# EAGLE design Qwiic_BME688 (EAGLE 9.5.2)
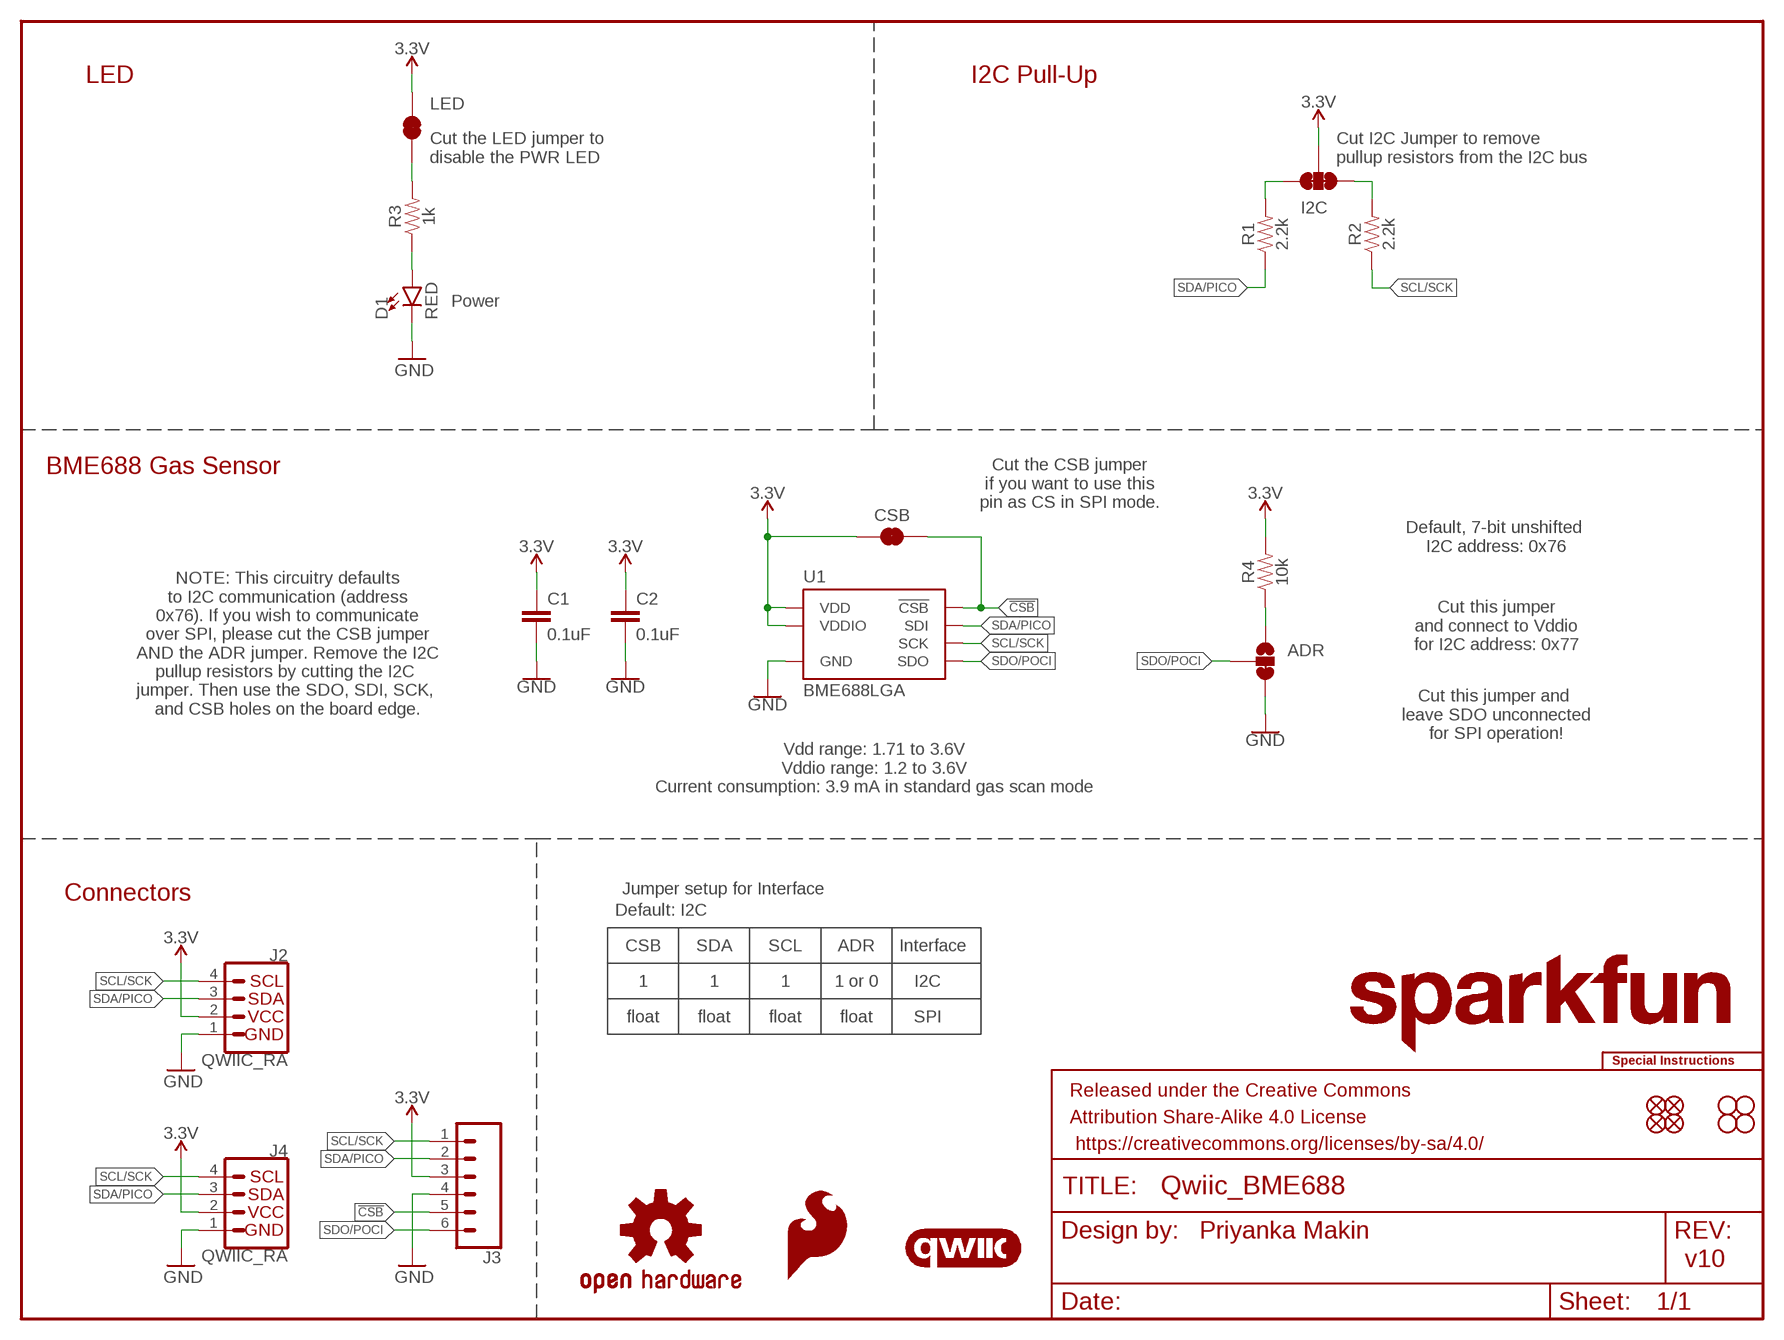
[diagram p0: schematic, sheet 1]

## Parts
ADR  JUMPER-SMT_3_1-NC_TRACE_SILK  [SMT-JUMPER_3_1-NC_TRACE_SILK]
C1  0.1uF  0.1UF-0603-100V-10%  [0603]
C2  0.1uF  0.1UF-0603-100V-10%  [0603]
CSB  JUMPER-SMT_2_NC_TRACE_SILK  [SMT-JUMPER_2_NC_TRACE_SILK]
D1  RED  LED-RED0603  [LED-0603]
FRAME1  FRAME-LETTER  [CREATIVE_COMMONS]
I2C  JUMPER-SMT_3_2-NC_TRACE_SILK  [SMT-JUMPER_3_2-NC_TRACE_SILK]
J2  QWIIC_RA  QWIIC_CONNECTORJS-1MM  [JST04_1MM_RA]
J3  CONN_06NO_SILK_NO_POP  [1X06_NO_SILK]
J4  QWIIC_RA  QWIIC_CONNECTORJS-1MM  [JST04_1MM_RA]
JP1  FIDUCIALUFIDUCIAL  [FIDUCIAL-MICRO]
JP2  FIDUCIALUFIDUCIAL  [FIDUCIAL-MICRO]
JP3  STAND-OFF  [STAND-OFF]
JP4  STAND-OFF  [STAND-OFF]
JP5  FIDUCIALUFIDUCIAL  [FIDUCIAL-MICRO]
JP6  FIDUCIALUFIDUCIAL  [FIDUCIAL-MICRO]
JP7  STAND-OFF  [STAND-OFF]
JP8  STAND-OFF  [STAND-OFF]
LED  JUMPER-SMT_2_NC_TRACE_SILK  [SMT-JUMPER_2_NC_TRACE_SILK]
LOGO1  SPECIAL_INSTRUCTIONS-ORDERING  [ORDERING_INSTRUCTIONS]
LOGO2  QWIIC_LOGO_5MM  [QWIIC_5MM]
LOGO3  SFE_LOGO_NAME.1_INCH  [SFE_LOGO_NAME_.1]
LOGO4  SFE_LOGO_FLAME.1_INCH  [SFE_LOGO_FLAME_.1]
LOGO5  OSHW-LOGOS  [OSHW-LOGO-S]
LOGO6  SFE_LOGO_NAME.1_INCH  [SFE_LOGO_NAME_.1]
R1  2.2k  2.2KOHM-0603-1/10W-1%  [0603]
R2  2.2k  2.2KOHM-0603-1/10W-1%  [0603]
R3  1k  1KOHM-0603-1/10W-1%  [0603]
R4  10k  10KOHM-0603-1/10W-1%  [0603]
U1  BME688LGA  [LGA_8PIN]

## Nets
3.3V: C1.1 C2.1 CSB.1 I2C.2 J2.2 J3.3 J4.2 LED.2 R4.2 U1.6(VDDIO) U1.8(VDD)
!CSB!: CSB.2 J3.5 U1.2(!CSB!)
GND: ADR.3 C1.2 C2.2 D1.C J2.1 J3.4 J4.1 U1.1(GND) U1.7(GND)
N$1: LED.1 R3.2
N$2: I2C.3 R1.2
N$3: D1.A R3.1
N$4: I2C.1 R2.2
N$5: ADR.1 R4.1
SCL/SCK: J2.4 J3.1 J4.4 R2.1 U1.4(SCK)
SDA/PICO: J2.3 J3.2 J4.3 R1.1 U1.3(SDI)
SDO/POCI: ADR.2 J3.6 U1.5(SDO)

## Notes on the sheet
- LED | I2C Pull-Up
- Cut the LED jumper to
  disable the PWR LED
- Cut I2C Jumper to remove 
  pullup resistors from the I2C bus
- Power
- BME688 Gas Sensor
- Cut the CSB jumper
  if you want to use this
  pin as CS in SPI mode.
- Default, 7-bit unshifted 
  I2C address: 0x76
- Cut this jumper
  and connect to Vddio
  for I2C address: 0x77
- NOTE: This circuitry defaults
  to I2C communication (address
  0x76). If you wish to communicate
  over SPI, please cut the CSB jumper
  AND the ADR jumper. Remove the I2C
  pullup resistors by cutting the I2C 
  jumper. Then use the SDO, SDI, SCK, 
  and CSB holes on the board edge.
- Cut this jumper and 
  leave SDO unconnected
  for SPI operation!
- Vdd range: 1.71 to 3.6V
  Vddio range: 1.2 to 3.6V
  Current consumption: 3.9 mA in standard gas scan mode
- Connectors | Jumper setup for Interface
- Default: I2C
- CSB | SDA | SCL | ADR | Interface
- 1 | 1 | 1 | 1 or 0 | I2C
- float | float | float | float | SPI
- Priyanka Makin
- v10

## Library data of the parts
ADR = SparkFun-Jumpers:JUMPER-SMT_3_1-NC_TRACE: Normally closed trace jumper (1 of 2 connections) This jumper has a trace between two pads so it's normally closed (NC). The other connection is normally open (NO). Use a razor knife to open the connection. For best results follow the IPC guidelines for cutting traces: Cutout at least 0.063 mm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
C1 C2 = SparkFun-Capacitors:0.1UF: 0.1µF ceramic capacitors; PROD_ID: CAP-08390
CSB LED = SparkFun-Jumpers:JUMPER-SMT_2_NC_TRACE: Normally closed trace jumper
D1 = SparkFun-LED:LED-RED: Red SMD LED; PROD_ID: DIO-00819
FRAME1 = SparkFun-Aesthetics:FRAME-LETTER: Schematic Frame - Letter
I2C = SparkFun-Jumpers:JUMPER-SMT_3_2-NC_TRACE: Normally closed trace jumper (2 of 2 connections) This jumper has a trace between all three pads so they are normally closed (NC). Use a razor knife to open the connection(s). For best results follow the IPC guidelines for cutting traces: Cutout at least 0.063 mm (0.005 in). Remove all loose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
J2 J4 = SparkFun-Connectors:QWIIC_CONNECTOR: SparkFun I2C Standard Qwiic Connector An SMD 1mm pitch JST connector makes it easy and quick (get it? Qwiic?) to connect I2C devices to each other. The Qwiic system enables fast and solderless connection between popular platforms and various sensors and actuators. We carry 200mm, 100mm, 50mm, and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; PROD_ID: CONN-13694; VALUE: QWIIC_RIGHT_ANGLE
J3 = SparkFun-Connectors:CONN_06: Multi connection point. Often used as Generic Header-pin footprint for 0.1 inch spaced/style header connections On any of the 0.1 inch spaced packages, you can populate with these: Break Away Headers - Straight (PRT-00116) Break Away Male Headers - Right Angle (PRT-00553) Female Headers (PRT-00115)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
JP1 JP2 JP5 JP6 = SparkFun-Aesthetics:FIDUCIAL: Fiducial Alignment Points
JP3 JP4 JP7 JP8 = SparkFun-Hardware:STAND-OFF: Stand Off
LOGO1 = SparkFun-Aesthetics:SPECIAL_INSTRUCTIONS: Special Ordering/Production Instructions Alert
LOGO2 = SparkFun-Aesthetics:QWIIC_LOGO: Qwiic Logos for placement on schematic and PCB. The 5.5mm silk logo is best for placing next to Qwiic connector.
LOGO3 LOGO6 = SparkFun-Aesthetics:SFE_LOGO_NAME: SparkFun Font Logo
LOGO4 = SparkFun-Aesthetics:SFE_LOGO_FLAME: SparkFun Flame Logo
LOGO5 = SparkFun-Aesthetics:OSHW-LOGO: Open-Source Hardware (OSHW) Logo
R1 R2 = SparkFun-Resistors:2.2KOHM: 2.2kΩ resistor; PROD_ID: RES-08272
R3 = SparkFun-Resistors:1KOHM: 1kΩ resistor; PROD_ID: RES-07856
R4 = SparkFun-Resistors:10KOHM: 10kΩ resistor; PROD_ID: RES-00824
U1 = BME688:BME688: BME688 gas sensor from Bosch.

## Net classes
1 power: width 0.203 mm

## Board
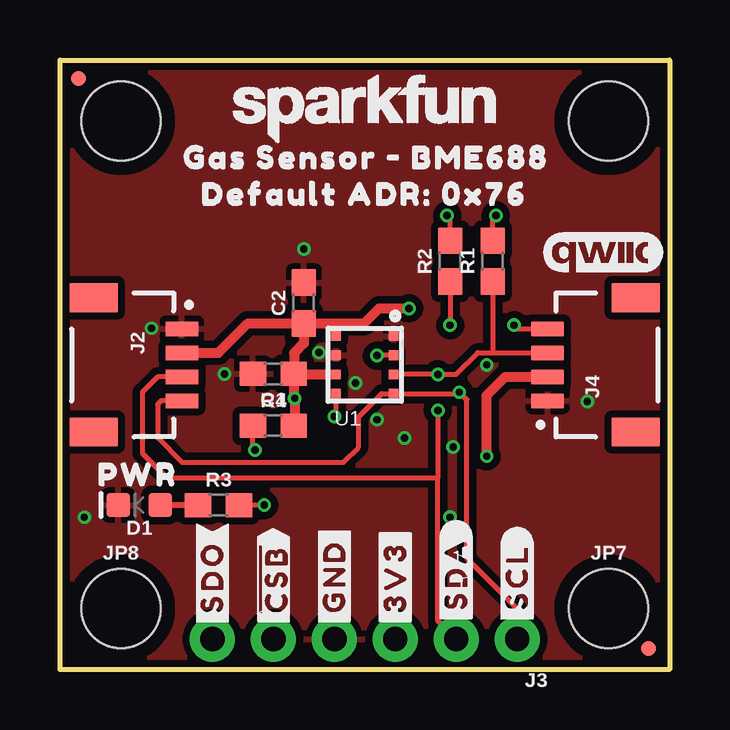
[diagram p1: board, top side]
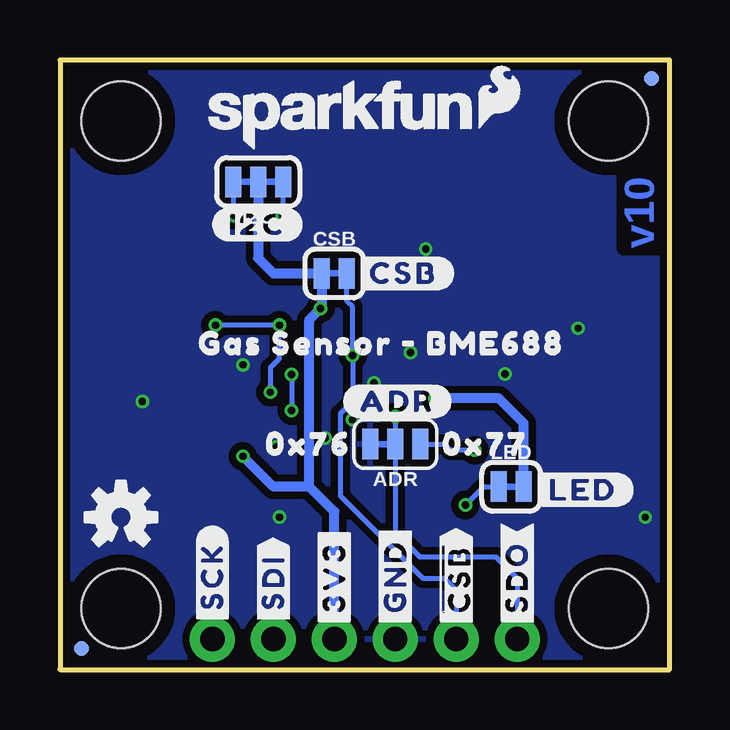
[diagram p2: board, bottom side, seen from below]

Size 25.4 x 25.4 mm. Coordinates in mm from the lower left corner, seen from the top.
Outline: 0,0 0,25.4 25.4,25.4 25.4,0 0,0
Copper layers (1*16): Top 0.035mm / dielectric 1.5mm / Bottom 0.035mm
Design rules "SparkFun-2-Layer-Minimum-JLCPCB": minimum track width 5mil, minimum drill 0.3mm, track to track 5mil, track to pad 5mil, pad to pad 5mil, via to via 5mil, smd to smd 5mil, copper to edge 7mil, drill to drill 7mil, minimum pad ring 5mil, minimum via ring 5mil, stop-mask expansion 2.5mil, vias tented up to drill 25mil, thermal gap 10mil

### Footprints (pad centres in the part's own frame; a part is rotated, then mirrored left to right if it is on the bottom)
SMT-JUMPER_3_1-NC_TRACE_SILK = smd 0.66 x 1.27: 1 -1.041,0; 2 0,0; 3 1.041,0
0603 = smd 1.1 x 1: 1 -0.85,0; 2 0.85,0
SMT-JUMPER_2_NC_TRACE_SILK = smd 0.66 x 1.27: 1 -0.521,0; 2 0.521,0
LED-0603 = smd 1 x 1: A -0.877,0; C 0.877,0
SMT-JUMPER_3_2-NC_TRACE_SILK = smd 0.66 x 1.27: 1 -1.041,0; 2 0,0; 3 1.041,0
JST04_1MM_RA = smd 0.6 x 1.35: 1 -1.5,0; 2 -0.5,0; 3 0.5,0; 4 1.5,0 | smd 1.2 x 2: NC1 2.8,-3.675; NC2 -2.8,-3.675
1X06_NO_SILK = drill 1.016 pad 1.88: 1 0,0; 2 2.54,0; 3 5.08,0; 4 7.62,0; 5 10.16,0; 6 12.7,0
FIDUCIAL-MICRO = smd 0.635 x 0.635: 1 0,0
STAND-OFF = hole 3.302: 0,0
LGA_8PIN = smd 0.4 x 0.4: 1 1.2,1.2; 2 1.2,0.4; 3 1.2,-0.4; 4 1.2,-1.2; 5 -1.2,-1.2; 6 -1.2,-0.4; 7 -1.2,0.4; 8 -1.2,1.2

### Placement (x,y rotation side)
ADR  11.43,9.4 180 bottom
C1  8.89,12.32 180 top
C2  10.16,15.28 90 top
CSB  13.97,16.51 0 bottom
D1  3.3,6.86 180 top
FRAME1  not placed on the board
I2C  17.14,20.32 180 bottom
J2  5.08,12.7 270 top
J3  19.05,1.27 180 top
J4  20.32,12.7 90 top
JP1  0.76,24.64 0 bottom
JP2  24.51,0.89 0 top
JP3  2.54,22.86 0 top
JP4  22.86,22.86 0 top
JP5  24.51,0.89 0 bottom
JP6  0.76,24.64 0 top
JP7  22.86,2.54 0 top
JP8  2.54,2.54 0 top
LED  6.6,7.62 0 bottom
LOGO1  not placed on the board
LOGO2  22.61,17.4 0 top
LOGO3  13.72,23.11 0 bottom
LOGO4  7.11,23.88 0 bottom
LOGO5  22.86,6.35 0 bottom
LOGO6  12.7,23.37 0 top
R1  18.03,17.02 90 top
R2  16.26,17.02 90 top
R3  6.6,6.86 0 top
R4  8.89,10.16 0 top
U1  12.7,12.7 0 top
U$1  [#GND#0]  11.43,1.65 90 bottom
U$2  [#SDO#0]  6.35,1.65 90 top
U$3  [#CSB#0]  13.21,16.51 0 bottom
U$5  [PWR0]  0.89,8.13 0 top
U$6  [#I2C#0]  19.05,18.54 0 bottom
U$7  [GAS_SENSOR_#_BME6880]  20.32,13.59 0 bottom
U$8  [#LED#0]  5.71,7.49 0 bottom
U$9  [0X760]  17.53,9.4 0 bottom
U$10  [GAS_SENSOR_#_BME6880]  4.45,21.34 0 top
U$11  [#ADR#0]  13.59,11.18 0 bottom
U$12  [DEFAULT_ADR#_0X760]  5.21,19.81 0 top
U$13  [0X770]  10.16,9.4 0 bottom
U$14  [#3V3#0]  13.97,1.65 90 top
U$15  [#3V3#0]  13.97,1.65 90 bottom
U$16  [#SDO#0]  6.35,1.65 90 bottom
U$19  [#SDI#0]  16.51,1.78 90 bottom
U$20  [#SCK#0]  19.05,1.78 90 bottom
U$21  [##CSB##0]  8.89,1.65 90 bottom
U$22  [##CSB##0]  8.89,1.65 90 top
U$33  [#GND#0]  11.43,1.65 90 top
U$35  [#SDA#0]  16.51,1.78 90 top
U$36  [#SCL#0]  19.05,1.78 90 top

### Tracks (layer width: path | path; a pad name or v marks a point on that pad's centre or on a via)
3.3V  (via drill 0.3)
  Top 0.406: J4.2 18.54,12.19 17.78,11.43 v17.78,8.89 | 9.76,12.3 C1.1 9.74,11.34 v9.78,11.3 9.78,10.2 R4.2 | 9.76,12.3 U1.6 | J2.2 6.6,13.2 7.83,14.43 C2.1 | C2.1 10.16,13.59 9.76,13.19 9.76,12.3 | C2.1 11.43,14.43 | 11.43,14.43 12.67,14.43 13.29,15.05 v14.54,15.05 | U1.8 11.5,14.36 11.43,14.43
  Bottom 0.406: v17.78,8.89 16.51,7.62 15.01,7.62 | I2C.2 17.14,17.14 16.51,16.51 CSB.1 14.48,16.51 14.48,15.11 v14.54,15.05 15.01,14.58 15.01,7.62 | J3.3 13.97,6.58 15.01,7.62 | LED.2 6.08,10.27 7.11,11.3 v9.78,11.3
!CSB!  (via drill 0.3)
  Top 0.203: U1.2 13.23,13.1 v13.21,13.08
  Bottom 0.203: CSB.2 13.45,15.35 13.21,15.11 v13.21,13.08 13.21,11.18 13.72,10.67 13.72,7.24 10.29,3.81 9.4,3.81 8.89,3.3 J3.5
GND  (via drill 0.3)
  other vias: 1.02,6.35 3.81,14.22 6.86,12.32 10.16,17.53 10.79,13.21 13.21,10.41 21.97,11.18 12.32,11.94 14.35,9.65 16.26,6.35 17.78,12.7 16.38,9.27
  pour Bottom (isolate 0.305): 0,0 0,25.4 25.4,25.4 25.4,0
  pour Top (isolate 0.305): 0,0 0,25.4 25.4,25.4 25.4,0
N$1  (via drill 0.3)
  Top 0.203: v8.51,6.86 R3.2
  Bottom 0.203: v8.51,6.86 7.75,7.62 LED.1
N$2  (via drill 0.3)
  Top 0.203: R1.2 18.03,18.8 v18.16,18.92
  Bottom 0.203: v18.16,18.92 18.16,20.3 I2C.3
N$3
  Top 0.254: R3.1 D1.A
N$4  (via drill 0.3)
  Top 0.203: R2.2 16.26,18.8 v16.13,18.92
  Bottom 0.203: v16.13,18.92 16.1,18.95 I2C.1
N$5  (via drill 0.3)
  Top 0.203: v8.13,9.14 8.04,9.23 R4.1
  Bottom 0.203: v8.13,9.14 9.14,9.14 9.4,9.4 ADR.1
SCL/SCK  (via drill 0.3)
  Top 0.203: 16.69,11.5 U1.4 13.4,11.5 12.45,10.54 12.45,9.27 11.81,8.64 5.08,8.64 4.06,9.65 4.06,11.05 4.21,11.2 J2.4 | 16.69,11.5 16.95,11.25 16.95,4.64 19.05,2.54 J3.1 | 16.69,11.5 v16.64,11.56 | v18.92,14.35 19.07,14.2 J4.4 | R2.1 v16.26,14.35
  Bottom 0.203: v16.64,11.56 16.64,12.57 16.26,12.95 v16.26,14.35 v18.92,14.35
SDA/PICO  (via drill 0.3)
  Top 0.203: U1.3 v15.75,12.3 16.49,12.3 17.4,13.21 18.03,13.21 | 18.03,13.21 J4.3 | R1.1 18.03,13.21 | v15.75,10.79 15.75,8 | J2.3 4.07,12.2 3.43,11.56 3.43,9.02 4.45,8 15.75,8 | J3.2 15.75,2.03 15.75,8
  Bottom 0.203: v15.75,12.3 v15.75,10.79
SDO/POCI  (via drill 0.3)
  Top 0.203: v11.43,10.54 11.5,10.61 U1.5
  Bottom 0.203: v11.43,10.54 ADR.2 11.43,5.71 10.41,4.7 7.24,4.7 6.35,3.81 J3.6

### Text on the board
Bottom: v10
Measures: Dimensions in inches
tDocu: 2 Layers / 1.6mm Thickness / HASL lead-free Finish | Priyanka Makin

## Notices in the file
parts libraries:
SparkFun-Resistors: Licensing: Creative Commons ShareAlike 4.0 International - https://creativecommons.org/licenses/by-sa/4.0
SparkFun-Aesthetics: Released under the Creative Commons Attribution Share-Alike 4.0 License
SparkFun-Aesthetics: https://creativecommons.org/licenses/by-sa/4.0
